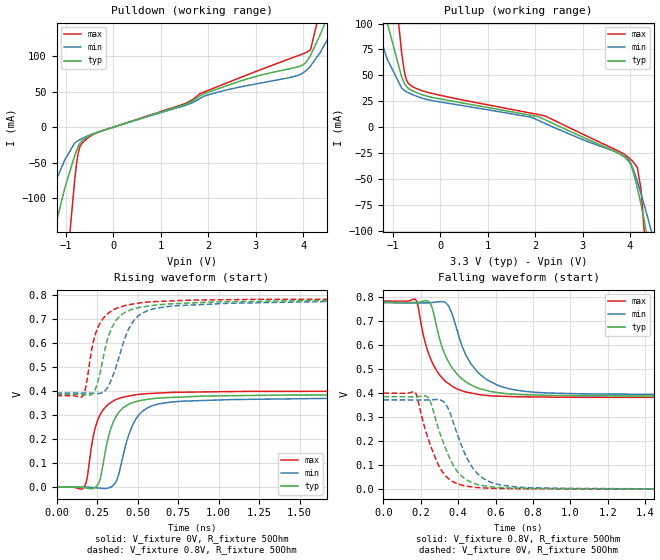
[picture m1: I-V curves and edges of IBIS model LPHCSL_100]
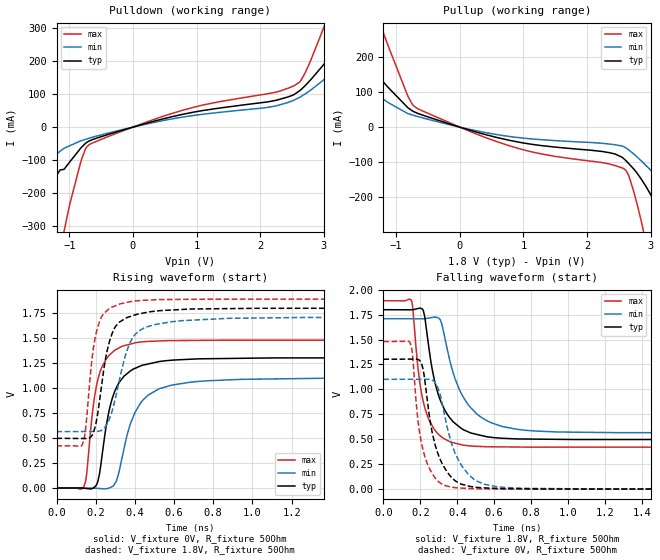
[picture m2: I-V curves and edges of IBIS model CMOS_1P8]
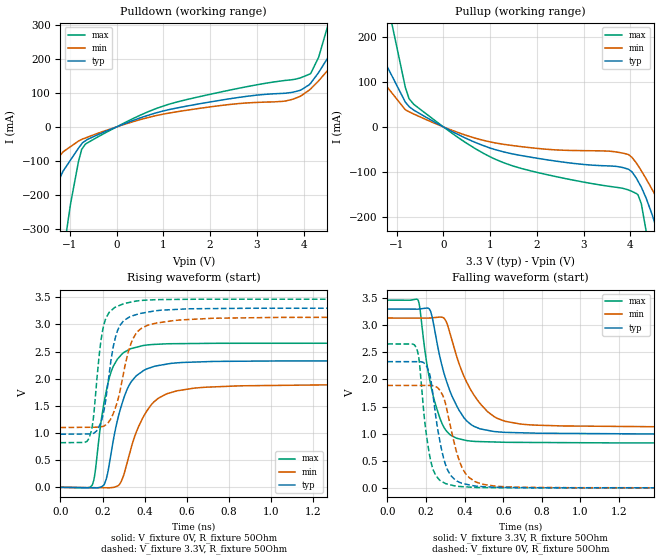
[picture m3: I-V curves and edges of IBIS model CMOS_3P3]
|Texas Instruments Incorporated
|Reference-Less 2-Differential or 5-Single-Ended Output
| PCIe Gen 1-6 Compliant Programmable BAW Clock Generator
| Marketing Part # : LMK3H0102
| Digital Voltage Range : 1.8V, 2.5V, 3.3V
| Package-type: RER
| #pins/pkg drawing : 16-pin TQFN
[IBIS Ver] 4.1
[File name] lmk3h0102.ibs
[File Rev] 1.0
[Date] 11/07/2023
[Source]
| Texas Instruments Incorporated.
| 12500 TI Blvd
| Dallas, TX -75243
[Notes] Revision History:
| Rev 1.0: 11/07/2023
| - Initial version of the model
| - Model generated from simulations in TISPICE/SPECTRE
| - C_comp although listed in numerical order of value are
| obtained from varying PVT conditions. For PVT conditions for
| each specific value refer the buffer description under
| respective [Model]. IBIS model user is responsible for using
| appropriate C_comp to simulate for Signal Integrity.
| - Warnings regarding combined Non-monotonicity of various models have been
| reviewed and considered minor and can be ignored.
|**** Modify the following if you use [Model Selector]*****************
| - Model names with a trailing _1p8 contain the model for
| 1.8V operation. Model names with a trailing _3p3 contain the model
| for 3.3V operation.
[Disclaimer]
| This model is designed as an aid for customers of Texas Instruments.
| TI and its licensors and suppliers make no warranties, either expressed
| or implied, with respect to this model, including the warranties of
| merchantability or fitness for a particular purpose. The model is
| provided solely on an "as is" basis. The entire risk as to its quality
| and performance is with the customer.
| This model is subject to change without notice. Texas Instruments
| Incorporated is not responsible for updating this model.
[Copyright]
(C) Copyright 2023 Texas Instruments Incorporated. All rights reserved.
[Component] LMK03H0102
[Manufacturer] Texas Instruments Incorporated
[Package] |RER (TQFN) 16-pin
| variable typ min max
R_pkg 0.3 0.25 0.35
L_pkg 0.5nH 0.4nH 0.6nH
C_pkg 0.13pF 0.1pF 0.16pF
| pin number (pin name) mapping to model name
[Pin] signal_name model_name R_pin L_pin C_pin
1  OE   oe   0.22752 0.46627n 0.11004p
2  FMT_ADDR gpi   0.2519  0.51198n 0.12793p
3  SCL   scl   0.23702 0.47768n 0.12641p
4  SDA   sda   0.2514  0.52409n 0.11517p
5  VDD   power   0.15234 0.32707n 0.25042p
6  NC   nc   NA   NA   NA
7  OUT0_N   output  0.31653 0.64547n 0.14401p
8  OUT0_P   output  0.30988 0.64858n 0.13114p
9  NC   nc   NA   NA   NA
10 VDDO_0   power   0.23544 0.47574n 0.12686p
11 OUT1_N   output  0.25227 0.51147n 0.12799p
12 OUT1_P   output  0.22848 0.46651n 0.10991p
13 VDDO_1   power   0.22172 0.45045n 0.10844p
14 VDD   power   0.26275 0.53341n 0.12873p
15 REF_CTRL ref_out 0.26507 0.53959n 0.12948p
16 VDD   power   0.21951 0.44923n 0.10861p
| Differential pin definition
| Use in differential output types, LP-HCSL, LVDS
[Diff Pin] inv_pin vdiff tdelay_typ tdelay_min tdelay_max
| The 'OUTx_P' pin is Diff_pin and the 'OUTx_N' pin is the inv_pin|
8 7 10m  0 0 0
12 11 10m 0 0 0
| Model Selectors
[Model Selector] output
LPHCSL_100 LP-HCSL with 100O output termination
LPHCSL_85 LP-HCSL with 85O output termination
CMOS_1P8 CMOS with 1.8V VDD
CMOS_2P5 CMOS with 2.5V VDD
CMOS_3P3 CMOS with 3.3V VDD
LVDS_1P8 LVDS with 1.8V VDD
LVDS_2P5 LVDS with 2.5V VDD
LVDS_3P3 LVDS with 3.3V VDD
[Model Selector] ref_out
REF_CLK_1P8 CMOS REF_OUT with 1.8V VDD
REF_CLK_2P5 CMOS REF_OUT with 2.5V VDD
REF_CLK_3P3 CMOS REF_OUT with 3.3V VDD
INPUT_PIN15_CTRL_1P8 ctrl input with 1.8V VDD
INPUT_PIN15_CTRL_2P5 ctrl input with 2.5V VDD
INPUT_PIN15_CTRL_3P3 ctrl input with 3.3V VDD
[Model Selector] oe
INPUT_PIN1_OE_PD_1P8 OE input with 75k pulldown with 1.8V VDD
INPUT_PIN1_OE_PD_2P5 OE input with 75k pulldown with 2.5V VDD
INPUT_PIN1_OE_PD_3P3 OE input with 75k pulldown with 3.3V VDD
INPUT_PIN1_OE_PU_1P8 OE input with 75k pullup with 1.8V VDD
INPUT_PIN1_OE_PU_2P5 OE input with 75k pullup with 2.5V VDD
INPUT_PIN1_OE_PU_3P3 OE input with 75k pullup with 3.3V VDD
[Model Selector] gpi
GPI_weakPD_1P8 general purpose input with weak pulldown with 1.8V VDD
GPI_weakPD_2P5 general purpose input with weak pulldown with 2.5V VDD
GPI_weakPD_3P3 general purpose input with weak pulldown with 3.3V VDD
GPI_HS_OE_PD_1P8 second OE with 75k pulldown with 1.8V VDD
GPI_HS_OE_PD_2P5 second OE with 75k pulldown with 2.5V VDD
GPI_HS_OE_PD_3P3 second OE with 75k pulldown with 3.3V VDD
[Model Selector] scl
INPUT_I2C_1P8 SCL input with 1.8V VDD
INPUT_I2C_2P5 SCL input with 2.5V VDD
INPUT_I2C_3P3 SCL input with 3.3V VDD
[Model Selector] sda
OUTPUT_I2C_1P8 SDA output  with 1.8V VDD
OUTPUT_I2C_2P5 SDA output  with 2.5V VDD
OUTPUT_I2C_3P3 SDA output  with 3.3V VDD
INPUT_I2C_1P8 I2C input with 1.8V VDD
INPUT_I2C_2P5 I2C input with 2.5V VDD
INPUT_I2C_3P3 I2C input with 3.3V VDD
| Models and submodels in the file (32): LPHCSL_100 (Output), LPHCSL_85 (Output), CMOS_1P8 (Output), CMOS_2P5 (Output), CMOS_3P3 (Output), LVDS_1P8 (Output), LVDS_2P5 (Output), LVDS_3P3 (Output), REF_CLK_1P8 (Output), REF_CLK_2P5 (Output), REF_CLK_3P3 (Output), INPUT_I2C_1P8 (Input), INPUT_I2C_2P5 (Input), INPUT_I2C_3P3 (Input), OUTPUT_I2C_1P8 (Open_drain), OUTPUT_I2C_2P5 (Open_drain), OUTPUT_I2C_3P3 (Open_drain), INPUT_PIN15_CTRL_1P8 (Input), INPUT_PIN15_CTRL_2P5 (Input), INPUT_PIN15_CTRL_3P3 (Input), INPUT_PIN1_OE_PD_1P8 (Input), INPUT_PIN1_OE_PD_2P5 (Input), INPUT_PIN1_OE_PD_3P3 (Input), INPUT_PIN1_OE_PU_1P8 (Input), INPUT_PIN1_OE_PU_2P5 (Input), INPUT_PIN1_OE_PU_3P3 (Input), GPI_HS_OE_PD_1P8 (Input), GPI_HS_OE_PD_2P5 (Input), GPI_HS_OE_PD_3P3 (Input), GPI_weakPD_1P8 (Input), GPI_weakPD_2P5 (Input), GPI_weakPD_3P3 (Input)
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[Model]   LPHCSL_100
Model_type   Output
Polarity   Non-Inverting
Vmeas = 0.375
Vref = 0
Cref = 2pF
Rref = 100000
|   typ   min   max
C_comp   2.5pF   2pF   3pF
[Voltage Range]   3.3   3.135   3.465
[Temperature Range]   45   125   -40
[Pullup Reference]   3.3   3.135   3.465
[Pulldown Reference]   -0   0   -0
[Power Clamp Reference]   3.3   3.135   3.465
[GND Clamp Reference]   0   0   0
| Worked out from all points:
|   slope of the pulldown table from 0 to 0.495 V, typ, clamps not added: 46.9 ohm
|   slope of the pullup table from 0 to 0.495 V, typ, clamps not added: 121 ohm
|   falling waveform, V_fixture 0.8V, R_fixture 50Ohm: 20-80 % time 134ps typ, 152ps min, 118ps max; typ from 0.778 V to 0.387 V
|   rising waveform, V_fixture 0V, R_fixture 50Ohm: 20-80 % time 98ps typ, 113ps min, 87.4ps max; typ from 0 V to 0.385 V
|   rising waveform, V_fixture 0.8V, R_fixture 50Ohm: 20-80 % time 109ps typ, 133ps min, 96ps max; typ from 0.387 V to 0.778 V
|   falling waveform, V_fixture 0V, R_fixture 50Ohm: 20-80 % time 119ps typ, 126ps min, 110ps max; typ from 0.385 V to 0 V
[Pulldown]
|   Voltage   I(typ)   I(min)   I(max)
-3.3V     -899.1mA   -528.2mA   -2.692A
-1.944V   -395.2mA   -213.5mA   -1.201A
-1.241V   -149.6mA   -80.86mA   -439.1mA
-1.023V   -85.09mA   -45.71mA   -224.9mA
-706.2mV  -22.59mA   -17.56mA   -27.46mA
-429mV    -9.629mA   -9.193mA   -10.32mA
3.977V    86.76mA    75.29mA    102.5mA
4.155V    100.7mA    85.73mA    108.6mA
4.363V    130.4mA    105.2mA    165.8mA
4.59V     167.8mA    132.6mA    261.3mA
4.907V    230.9mA    176.3mA    408.7mA
6.6V      624.2mA    482.1mA    1.302A
[Pullup]
|   Voltage   I(typ)   I(min)   I(max)
-3.3V     597.5mA    427.6mA    1.347A
-1.617V   206.2mA    137.9mA    457.2mA
-1.112V   99.56mA    64.93mA    204.4mA
-815.1mV  48.52mA    37.71mA    71.73mA
-735.9mV  40.7mA     34.8mA     49.01mA
-627mV    36.08mA    32.22mA    40.36mA
2.095V    9.633mA    5.938mA    11.89mA
3.828V    -27.21mA   -26.75mA   -24.82mA
4.155V    -59.05mA   -52.46mA   -39.3mA
4.372V    -108mA     -87.23mA   -147.2mA
4.491V    -142.5mA   -107.7mA   -240.8mA
6.6V      -930.7mA   -594.1mA   -2.541A
[Ramp]
R_load = 50
|   typ   min   max
dV/dt_r   0.230932/9.7996e-11   0.222863/1.12745e-10   0.239773/8.73447e-11
dV/dt_f   0.234814/1.33534e-10   0.230538/1.51007e-10   0.241163/1.17227e-10
[Falling Waveform]
V_fixture = 0.8V
V_fixture_min = 0.8V
V_fixture_max = 0.8V
R_fixture = 50Ohm
C_fixture = 0F
|   Time   V(typ)   V(min)   V(max)
0s        777.9mV    775.9mV    783.1mV
173.3ps   777.2mV    775.5mV    788mV
220.1ps   783.6mV    775.4mV    620.1mV
250.2ps   773.8mV    776.2mV    547.1mV
335.1ps   549.9mV    774.8mV    446.8mV
438.6ps   448mV      562.4mV    405mV
518.4ps   417.6mV    476.5mV    392.7mV
702.4ps   395.1mV    413.2mV    384.9mV
1.074ns   389.2mV    396.6mV    382.4mV
5ns       386.6mV    391.7mV    381.2mV
[Rising Waveform]
V_fixture = 0V
V_fixture_min = 0V
V_fixture_max = 0V
R_fixture = 50Ohm
C_fixture = 0F
|   Time   V(typ)   V(min)   V(max)
0s        187uV      283.4uV    113.6uV
167.8ps   -1.962mV   152.4uV    -1.11mV
186.3ps   -3.82mV    138uV      30.16mV
245.8ps   3.068mV    -2.748mV   262.6mV
341.6ps   256.3mV    2.698mV    355.1mV
377.6ps   305.6mV    40.1mV     367.7mV
487.3ps   355.7mV    280.9mV    384.7mV
627.4ps   370.6mV    346.4mV    391.7mV
1.074ns   380.6mV    364.6mV    397.9mV
5ns       385.1mV    371.7mV    399.7mV
[Rising Waveform]
V_fixture = 0.8V
V_fixture_min = 0.8V
V_fixture_max = 0.8V
R_fixture = 50Ohm
C_fixture = 0F
|   Time   V(typ)   V(min)   V(max)
0s        386.6mV    391.7mV    381.2mV
164.7ps   385.2mV    391.9mV    382.7mV
237.3ps   404.2mV    390.3mV    631.1mV
296.4ps   565.9mV    399.4mV    708.7mV
323.7ps   635.2mV    426.7mV    726.5mV
370.6ps   697.3mV    507.6mV    744.7mV
438.6ps   732.6mV    649.3mV    758.7mV
518.4ps   749.1mV    720.2mV    767.6mV
1.074ns   771.9mV    765.9mV    780.6mV
5ns       777.9mV    775.8mV    783.1mV
[Falling Waveform]
|Gnd
V_fixture = 0V
V_fixture_min = 0V
V_fixture_max = 0V
R_fixture = 50Ohm
C_fixture = 0F
|   Time   V(typ)   V(min)   V(max)
0s        385.1mV    371.8mV    399.8mV
170.6ps   384.5mV    371.5mV    402.3mV
245.8ps   373.7mV    371.8mV    194.7mV
322.9ps   189mV      363.7mV    64.61mV
349.3ps   138.1mV    330.6mV    43.25mV
400.4ps   68.64mV    217.6mV    21.6mV
487.3ps   22.89mV    78.43mV    7.784mV
592ps     8.424mV    24.03mV    3.782mV
783.6ps   3.06mV     6.308mV    1.849mV
5ns       186.4uV    283.2uV    112.6uV
[Model]   CMOS_1P8
Model_type   Output
Polarity   Non-Inverting
Vmeas = 0.9
Vref = 0
Cref = 5pF
Rref = 100000
|   typ   min   max
C_comp   2.5pF   2pF   3pF
[Voltage Range]   1.8   1.71   1.89
[Temperature Range]   45   125   -40
[Pullup Reference]   1.8   1.71   1.89
[Pulldown Reference]   -0   0   0
[Power Clamp Reference]   1.8   1.71   1.89
[GND Clamp Reference]   0   0   0
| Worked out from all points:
|   slope of the pulldown table from 0 to 0.27 V, typ, clamps not added: 18.4 ohm
|   slope of the pullup table from 0 to 0.27 V, typ, clamps not added: 18.6 ohm
|   falling waveform, V_fixture 1.8V, R_fixture 50Ohm: 20-80 % time 106ps typ, 148ps min, 73.6ps max; typ from 1.8 V to 0.497 V
|   rising waveform, V_fixture 0V, R_fixture 50Ohm: 20-80 % time 87.7ps typ, 117ps min, 65ps max; typ from 0 V to 1.3 V
|   rising waveform, V_fixture 1.8V, R_fixture 50Ohm: 20-80 % time 71.3ps typ, 95.2ps min, 54ps max; typ from 0.497 V to 1.8 V
|   falling waveform, V_fixture 0V, R_fixture 50Ohm: 20-80 % time 89.4ps typ, 114ps min, 65.3ps max; typ from 1.3 V to 0 V
[Pulldown]
|   Voltage   I(typ)   I(min)   I(max)
-3.3V     -896.9mA   -527.2mA   -2.683A
-2.241V   -526.9mA   -267.7mA   -1.551A
-2.191V   -508.4mA   -289.9mA   -1.495A
-1.082V   -127.7mA   -63.86mA   -315.5mA
-815.1mV  -62.43mA   -41.12mA   -102.2mA
-686.4mV  -41.63mA   -33.4mA    -52.76mA
2.541V    99.48mA    82.36mA    125.9mA
2.709V    125.6mA    100.5mA    164.5mA
2.996V    188.7mA    142.4mA    299.5mA
3.561V    323.4mA    235.3mA    600.7mA
3.947V    417.7mA    301.4mA    813.4mA
6.6V      1.096A     805.1mA    2.285A
[Pullup]
|   Voltage   I(typ)   I(min)   I(max)
-3.3V     611.7mA    427.2mA    1.367A
-2.538V   426.9mA    291.3mA    957.8mA
-1.934V   287.1mA    190.5mA    642.4mA
-1.181V   124.8mA    77.46mA    259.7mA
-726mV    44.5mA     33.75mA    61.01mA
778.8mV   -37.57mA   -26.54mA   -53.2mA
2.571V    -88.86mA   -55.28mA   -117.9mA
2.927V    -169.3mA   -109.4mA   -330.8mA
3.184V    -257.6mA   -158.6mA   -591.5mA
3.373V    -327.8mA   -199.7mA   -797.2mA
3.749V    -470.9mA   -285.1mA   -1.217A
6.6V      -1.605A    -995.6mA   -4.458A
[Ramp]
R_load = 50
|   typ   min   max
dV/dt_r   0.781598/8.7657e-11   0.660933/1.16255e-10   0.887697/6.50233e-11
dV/dt_f   0.781477/1.06092e-10   0.686978/1.47193e-10   0.880919/7.36326e-11
[Falling Waveform]
V_fixture = 1.8V
V_fixture_min = 1.71V
V_fixture_max = 1.89V
R_fixture = 50Ohm
C_fixture = 0F
|   Time   V(typ)   V(min)   V(max)
0s        1.799V     1.709V     1.889V
150.8ps   1.798V     1.709V     1.895V
188.7ps   1.812V     1.708V     1.191V
213.7ps   1.799V     1.708V     896.2mV
264.6ps   1.199V     1.721V     633.7mV
302.4ps   921mV      1.711V     543.9mV
432.9ps   597mV      922.5mV    441mV
564.2ps   524.2mV    682.8mV    425.2mV
821.3ps   501.8mV    582.9mV    421.8mV
5ns       496.9mV    564.2mV    421.2mV
[Rising Waveform]
V_fixture = 0V
V_fixture_min = 0V
V_fixture_max = 0V
R_fixture = 50Ohm
C_fixture = 0F
|   Time   V(typ)   V(min)   V(max)
0s        126.1uV    4.936uV    54.96uV
138.1ps   -1.48mV    25.69uV    10.31mV
152.7ps   -4.894mV   27.89uV    123.8mV
201.1ps   22.94mV    -2.653mV   993.1mV
231.8ps   314.9mV    -6.633mV   1.21V
287.3ps   913mV      17.76mV    1.361V
406.5ps   1.202V     775.5mV    1.454V
530.4ps   1.266V     996mV      1.471V
944ps     1.297V     1.087V     1.478V
5ns       1.303V     1.102V     1.48V
[Rising Waveform]
V_fixture = 1.8V
V_fixture_min = 1.71V
V_fixture_max = 1.89V
R_fixture = 50Ohm
C_fixture = 0F
|   Time   V(typ)   V(min)   V(max)
0s        496.9mV    564.2mV    421.2mV
132.7ps   495mV      564.3mV    438.2mV
149ps     494.8mV    564.3mV    603.2mV
194.3ps   591.6mV    564.3mV    1.473V
246.9ps   1.255V     604.9mV    1.756V
297.2ps   1.602V     869.5mV    1.82V
383.1ps   1.72V      1.483V     1.866V
503.3ps   1.769V     1.635V     1.882V
879.1ps   1.794V     1.697V     1.888V
5ns       1.799V     1.709V     1.889V
[Falling Waveform]
|Gnd
V_fixture = 0V
V_fixture_min = 0V
V_fixture_max = 0V
R_fixture = 50Ohm
C_fixture = 0F
|   Time   V(typ)   V(min)   V(max)
0s        1.303V     1.102V     1.48V
144.7ps   1.304V     1.102V     1.469V
155.4ps   1.304V     1.102V     1.383V
183ps     1.303V     1.102V     761.4mV
201.1ps   1.28V      1.102V     513.3mV
279.1ps   451.2mV    1.072V     114.9mV
364.2ps   128mV      488mV      22.27mV
490.8ps   21.25mV    97.91mV    4.166mV
682.1ps   4.966mV    14.37mV    1.052mV
5ns       126.6uV    4.936uV    55.13uV
[Model]   CMOS_3P3
Model_type   Output
Polarity   Non-Inverting
Vmeas = 1.65
Vref = 0
Cref = 5pF
Rref = 100000
|   typ   min   max
C_comp   2.5pF   2pF   3pF
[Voltage Range]   3.3   3.135   3.465
[Temperature Range]   45   125   -40
[Pullup Reference]   3.3   3.135   3.465
[Pulldown Reference]   0   0   -0
[Power Clamp Reference]   3.3   3.135   3.465
[GND Clamp Reference]   0   0   0
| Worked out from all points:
|   slope of the pulldown table from 0 to 0.495 V, typ, clamps not added: 19.1 ohm
|   slope of the pullup table from 0 to 0.495 V, typ, clamps not added: 19.1 ohm
|   falling waveform, V_fixture 3.3V, R_fixture 50Ohm: 20-80 % time 121ps typ, 158ps min, 85.3ps max; typ from 3.3 V to 0.977 V
|   rising waveform, V_fixture 0V, R_fixture 50Ohm: 20-80 % time 90.5ps typ, 118ps min, 68.3ps max; typ from 0 V to 2.33 V
|   rising waveform, V_fixture 3.3V, R_fixture 50Ohm: 20-80 % time 58.7ps typ, 79.1ps min, 44.5ps max; typ from 0.977 V to 3.3 V
|   falling waveform, V_fixture 0V, R_fixture 50Ohm: 20-80 % time 67.1ps typ, 82.6ps min, 51.7ps max; typ from 2.33 V to 0 V
[Pulldown]
|   Voltage   I(typ)   I(min)   I(max)
-3.3V     -898.7mA   -527.4mA   -2.7A
-2.221V   -519.6mA   -296.6mA   -1.531A
-1.34V    -191.5mA   -106.5mA   -555.6mA
-1.142V   -129.2mA   -72.78mA   -373.2mA
-745.8mV  -49.76mA   -36.85mA   -65.83mA
-448.8mV  -25.8mA    -21.14mA   -33.01mA
1.115V    50.53mA    40.45mA    66.37mA
3.947V    108.3mA    91.01mA    144.5mA
4.155V    128.4mA    111.8mA    156.8mA
4.739V    250.7mA    200.8mA    399.6mA
4.887V    285.3mA    225.4mA    475.8mA
6.6V      704.3mA    529.6mA    1.403A
[Pullup]
|   Voltage   I(typ)   I(min)   I(max)
-3.3V     609.5mA    425.1mA    1.365A
-1.934V   285.8mA    189.3mA    641.1mA
-1.716V   237.9mA    154.8mA    529.2mA
-627mV    36.8mA     28.27mA    49.5mA
1.304V    -55.73mA   -38.73mA   -79.83mA
3.67V     -87.1mA    -54.99mA   -133.3mA
4.125V    -113mA     -79.48mA   -147.3mA
4.234V    -133.3mA   -96.94mA   -170mA
4.333V    -156.6mA   -114.2mA   -227.9mA
4.61V     -243.3mA   -166.9mA   -459.3mA
5.501V    -579.3mA   -365.4mA   -1.435A
6.6V      -986.2mA   -624.5mA   -2.635A
[Ramp]
R_load = 50
|   typ   min   max
dV/dt_r   1.39742/9.02681e-11   1.13405/1.1812e-10   1.59328/6.82276e-11
dV/dt_f   1.39297/1.20871e-10   1.2199/1.57289e-10   1.58542/8.50419e-11
[Falling Waveform]
V_fixture = 3.3V
V_fixture_min = 3.135V
V_fixture_max = 3.465V
R_fixture = 50Ohm
C_fixture = 0F
|   Time   V(typ)   V(min)   V(max)
0s        3.299V     3.134V     3.464V
160.1ps   3.298V     3.133V     3.46V
217.5ps   3.302V     3.133V     2.028V
252.4ps   2.774V     3.145V     1.506V
303.9ps   1.995V     3.077V     1.06V
360.2ps   1.507V     2.413V     914.7mV
413.1ps   1.229V     1.935V     871mV
553.5ps   1.04V      1.313V     846.5mV
764.4ps   1.01V      1.157V     837.5mV
5ns       977.3mV    1.101V     821.7mV
[Rising Waveform]
V_fixture = 0V
V_fixture_min = 0V
V_fixture_max = 0V
R_fixture = 50Ohm
C_fixture = 0F
|   Time   V(typ)   V(min)   V(max)
0s        73.97uV    5.123uV    -3.854uV
152.2ps   -8.255mV   -5.765mV   49.67mV
164.6ps   -8.931mV   -6.233mV   270.8mV
205.6ps   38.59mV    -7.787mV   1.523V
247.3ps   776.8mV    -2.972mV   2.191V
304.2ps   1.675V     267.4mV    2.489V
393ps     2.143V     1.289V     2.61V
509.4ps   2.271V     1.726V     2.642V
855.8ps   2.321V     1.868V     2.651V
5ns       2.329V     1.89V      2.655V
[Rising Waveform]
V_fixture = 3.3V
V_fixture_min = 3.135V
V_fixture_max = 3.465V
R_fixture = 50Ohm
C_fixture = 0F
|   Time   V(typ)   V(min)   V(max)
0s        977.3mV    1.101V     821.6mV
137.9ps   982.6mV    1.105V     925.1mV
156.5ps   994mV      1.106V     1.273V
193.7ps   1.212V     1.113V     2.728V
228ps     1.977V     1.195V     3.195V
271.3ps   2.883V     1.587V     3.332V
320.3ps   3.116V     2.461V     3.397V
358.2ps   3.176V     2.824V     3.428V
724.8ps   3.29V      3.112V     3.462V
5ns       3.299V     3.134V     3.464V
[Falling Waveform]
|Gnd
V_fixture = 0V
V_fixture_min = 0V
V_fixture_max = 0V
R_fixture = 50Ohm
C_fixture = 0F
|   Time   V(typ)   V(min)   V(max)
0s        2.329V     1.89V      2.655V
150.4ps   2.328V     1.89V      2.583V
166.1ps   2.328V     1.89V      2.313V
202.6ps   2.251V     1.89V      975.1mV
235.3ps   1.742V     1.886V     356.5mV
285.2ps   638.5mV    1.718V     109.8mV
347.8ps   159.1mV    810.6mV    37.29mV
423.4ps   55.01mV    190.2mV    14.68mV
590.1ps   8.116mV    24.07mV    2.071mV
5ns       75.19uV    5.123uV    -3.521uV
